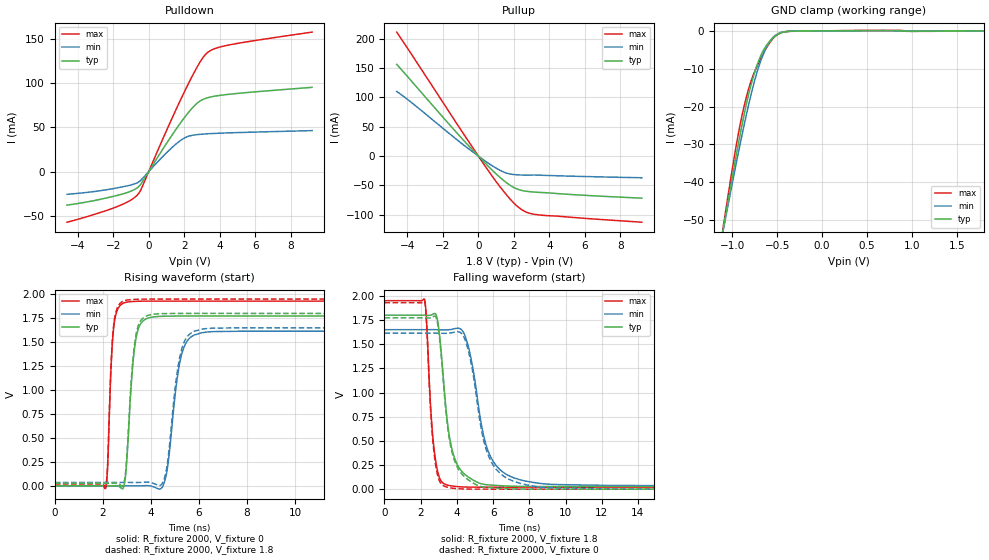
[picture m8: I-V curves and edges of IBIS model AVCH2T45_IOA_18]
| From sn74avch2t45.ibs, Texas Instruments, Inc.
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[Model]   AVCH2T45_IOA_18
Model_type  I/O
Vinl=0.5775
Vinh=1.2675
Enable   Active-Low
Vref =   0
Rref =   2000
Cref =   15p
Vmeas =   0.9
| variable   typ   min   max
C_comp   5.26pF   4.50pF   5.87pF
| C_pullup   4.77pF   3.53pF   6.89pF
| C_pulldown   4.67pF   4.09pF   5.05pF
| C_tri-state   5.26pF   4.50pF   5.87pF
[Temperature Range]   40   100   -40
| Ambient temperature   25   85   -40
[Voltage range]   1.8   1.65   1.95
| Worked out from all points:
|   slope of the pulldown table from 0 to 0.27 V, typ, clamps not added: 30.8 ohm
|   slope of the pullup table from 0 to 0.27 V, typ, clamps not added: 31.4 ohm
|   GND clamp passes 1 mA (typ) near -0.49 V on its own axis
|   rising waveform, R_fixture 2000, V_fixture 0: 20-80 % time 290ps typ, 449ps min, 186ps max; typ from 0 V to 1.77 V
|   falling waveform, R_fixture 2000, V_fixture 1.8: 20-80 % time 651ps typ, 999ps min, 376ps max; typ from 1.8 V to 0.027 V
|   rising waveform, R_fixture 2000, V_fixture 1.8: 20-80 % time 287ps typ, 440ps min, 184ps max; typ from 0.027 V to 1.8 V
|   falling waveform, R_fixture 2000, V_fixture 0: 20-80 % time 653ps typ, 998ps min, 362ps max; typ from 1.77 V to 0 V
[GND Clamp]
| AVCH2T45_IOA_18
|   Voltage   I(typ)   I(min)   I(max)
-4.6V     -599.6mA   -548.2mA   -664.6mA
-1.1V     -52.38mA   -52.81mA   -51.88mA
-1.075V   -48.92mA   -49.68mA   -47.98mA
-930mV    -29.69mA   -32.08mA   -27.04mA
-830mV    -18.1mA    -20.91mA   -16.44mA
-755mV    -11.37mA   -13.59mA   -11.08mA
-675mV    -6.227mA   -7.502mA   -6.966mA
-595mV    -3.153mA   -3.319mA   -3.603mA
-520mV    -1.409mA   -1.191mA   -1.426mA
-440mV    -417.5uA   -333.3uA   -376.2uA
-275mV    -54.37uA   -36.84uA   -89.06uA
1.8V      919.2pA    1.999uA    -415.8nA
[Pulldown]
| AVCH2T45_IOA_18
|   Voltage   I(typ)   I(min)   I(max)
-4.6V     -37.94mA   -25.73mA   -57.23mA
-1.8V     -27.09mA   -18.52mA   -39.79mA
-1.045V   -22.5mA    -15.36mA   -32.7mA
-590mV    -17.44mA   -12.06mA   -25.35mA
-395mV    -12.81mA   -8.801mA   -18.52mA
1.005V    31.93mA    21.31mA    46.48mA
1.825V    55.97mA    35.61mA    82.46mA
2.68V     76.51mA    41.68mA    116.5mA
3.045V    81.48mA    42.38mA    128.6mA
3.34V     83.6mA     42.77mA    135mA
4.575V    87.52mA    43.81mA    143.4mA
9.2V      95.24mA    46.32mA    157.7mA
[Pullup]
| AVCH2T45_IOA_18
|   Voltage   I(typ)   I(min)   I(max)
-4.6V     156.3mA    109.9mA    211.2mA
-3.695V   125.1mA    89.45mA    169.9mA
-1.245V   40.55mA    28.8mA     56.51mA
535mV     -16.77mA   -11.6mA    -23.84mA
1.065V    -32.16mA   -21.66mA   -46.14mA
1.49V     -43.16mA   -27.88mA   -62.67mA
1.925V    -52.28mA   -31.05mA   -77.72mA
2.305V    -57.27mA   -32.09mA   -88.3mA
2.77V     -60.1mA    -32.26mA   -96.25mA
3.4V      -61.74mA   -32.39mA   -100.1mA
9.2V      -71.58mA   -36.85mA   -112.5mA
[Ramp]
| AVCH2T45_IOA_18
| variable   typ   min   max
dV/dt_r   1.08/3.02E-10   0.99/4.61E-10   1.17/1.95E-10
dV/dt_f   1.07/6.57E-10   0.98/1.01E-09   1.17/3.80E-10
R_load = 2000
[Rising Waveform]
| AVCH2T45_IOA_18
R_fixture =   2000
C_fixture =   0
L_fixture =   0
V_fixture =   0
V_fixture_min = 0
V_fixture_max = 0
|   Time   V(typ)   V(min)   V(max)
0s        21.35nV    98.25nV    665.6pV
2.13ns    39.1uV     -109.8nV   -19.35mV
2.455ns   607.4uV    -20.47uV   1.66V
2.965ns   158.7mV    12.38uV    1.916V
3.365ns   1.517V     -172.4uV   1.926V
4.005ns   1.76V      -927.5uV   1.929V
4.615ns   1.771V     87.26mV    1.929V
5.33ns    1.772V     1.415V     1.929V
6.095ns   1.773V     1.597V     1.929V
34.99ns   1.772V     1.614V     1.929V
[Falling Waveform]
| AVCH2T45_IOA_18
R_fixture =   2000
C_fixture =   0
L_fixture =   0
V_fixture =   1.8
V_fixture_min = 1.65
V_fixture_max = 1.95
|   Time   V(typ)   V(min)   V(max)
0s        1.8V       1.65V      1.95V
2.215ns   1.8V       1.65V      1.964V
2.755ns   1.818V     1.65V      391.2mV
3.02ns    1.628V     1.649V     128.1mV
3.46ns    718.6mV    1.648V     43.78mV
3.825ns   346.5mV    1.659V     30.37mV
4.385ns   162.1mV    1.614V     22.62mV
5.72ns    44.71mV    397.5mV    20.42mV
7.445ns   28.88mV    99.42mV    20.34mV
34.99ns   27.01mV    36.05mV    20.32mV
[Rising Waveform]
| AVCH2T45_IOA_18
R_fixture =   2000
C_fixture =   0
L_fixture =   0
V_fixture =   1.8
V_fixture_min = 1.65
V_fixture_max = 1.95
|   Time   V(typ)   V(min)   V(max)
0s        27.01mV    36.05mV    20.32mV
2.13ns    27.05mV    36.05mV    1.244mV
2.455ns   27.62mV    36.03mV    1.685V
2.965ns   191.4mV    36.06mV    1.937V
3.365ns   1.554V     35.88mV    1.947V
3.995ns   1.787V     35.5mV     1.95V
4.605ns   1.798V     120mV      1.95V
5.31ns    1.8V       1.452V     1.95V
6.065ns   1.8V       1.633V     1.95V
34.99ns   1.8V       1.65V      1.95V
[Falling Waveform]
| AVCH2T45_IOA_18
R_fixture =   2000
C_fixture =   0
L_fixture =   0
V_fixture =   0
V_fixture_min = 0
V_fixture_max = 0
|   Time   V(typ)   V(min)   V(max)
0s        1.772V     1.614V     1.929V
2.215ns   1.772V     1.614V     1.943V
2.75ns    1.79V      1.615V     355.8mV
3.015ns   1.606V     1.614V     94.97mV
3.425ns   746.6mV    1.613V     22.96mV
3.785ns   344.6mV    1.621V     9.7mV
4.37ns    137mV      1.581V     2.031mV
5.71ns    16.98mV    360.8mV    85.26uV
7.48ns    1.537mV    60.76mV    10.27uV
34.99ns   454nV      473.3nV    331.7nV
